// generates a signal build up by the specified function type. v1.6
FUNCTION_BLOCK FB_FunctionGenerator
VAR_INPUT
	bEnable		: BOOL 	:= TRUE;	// set TRUE to generate the specified signal; set FALSE to reset the signal buffer
	fFrequency	: LREAL := 1000;	// in [Hz]
	fAmplitude	: LREAL := 1;
	fOffset		: LREAL	:= 0;	
	nDutyCycle	: UINT 	:= 50;		// in [%] (for pulse function)
	eFunction	: E_FunctionType := E_FunctionType.Sine;	
END_VAR
VAR_IN_OUT
	aSignal		: ARRAY[1..cOversamples] OF LREAL;
END_VAR
VAR_OUTPUT
	bError		: BOOL;
END_VAR

VAR
	bInit						: BOOL := TRUE;
	fbGetTaskIdx				: GETCURTASKINDEX;
	
	fLastFrequency				: LREAL;		// in [Hz]
	fLastAmplitude				: LREAL;
	fLastOffset					: LREAL;
	nLastDutyCycle				: UINT;
	eLastFunction				: E_FunctionType;
	
	nSamples					: UDINT;
	fCycleTime					: LREAL;		// in [s]
	fDelta						: LREAL;		// amplitude delta per sample
	fPhase						: LREAL;		// in [°]
	nSign						: INT := 1;		// 1 or -1
	fLastSignalValue			: LREAL;		// amplitude
	fPeriod						: LREAL;		// in [s]
	fAngularIncrement			: LREAL;		// in [°]
	fAngularIncrementPerCycle	: LREAL;		// in [°]
	fAngularIncrementPerSample	: LREAL;		// in [°]
	(* for modulated signal (carrier signal without offset) *)
	fCarrierFrequency					: LREAL := 500;	// in [Hz] (sine)
	fCarrierAmplitude					: LREAL := 1;
	fCarrierPeriod						: LREAL;		// in [s]
	fCarrierAngularIncrement			: LREAL;		// in [°]
	fCarrierAngularIncrementPerCycle	: LREAL;		// in [°]
	fCarrierAngularIncrementPerSample	: LREAL;		// in [°]
				
END_VAR

IF bEnable THEN
	IF fLastFrequency <> fFrequency THEN
		bInit := TRUE; // For automatic initializing
		fLastFrequency := fFrequency;
	END_IF
	IF fLastAmplitude <> fAmplitude THEN
		bInit := TRUE; // For automatic initializing
		fLastAmplitude := fAmplitude;
	END_IF
	IF fLastOffset <> fOffset THEN
		bInit := TRUE; // For automatic initializing
		fLastOffset := fOffset;
	END_IF
	IF nLastDutyCycle <> nDutyCycle THEN
		bInit := TRUE; // For automatic initializing
		nLastDutyCycle := nDutyCycle;
	END_IF
	IF eLastFunction <> eFunction THEN
		bInit := TRUE; // For automatic initializing
		eLastFunction := eFunction;
	END_IF
	IF bInit THEN
		// Get task info	
		fbGetTaskIdx();
		fCycleTime := UDINT_TO_LREAL(TwinCAT_SystemInfoVarList._TaskInfo[fbGetTaskIdx.index].CycleTime) (*100ns*) / (10.0 * 1000.0 * 1000.0);	
		fLastSignalValue := 0;
		nSign := 1;
		fAngularIncrement := 0;
		// Flush out old data
		MEMSET(ADR(aSignal), 0, SIZEOF(aSignal));
		IF fFrequency > 0 AND fCycleTime > 0 THEN		
			// Calculate period, increments per plc cycle, increment per oversample
			IF cOversamples > 0 THEN			
				IF eFunction = E_FunctionType.Sine THEN
					fPeriod := 1/fFrequency;
					fAngularIncrementPerCycle := 360*(fCycleTime/fPeriod);
					fAngularIncrementPerSample := fAngularIncrementPerCycle/cOversamples;
					// no phase adjustment
					bInit := FALSE;	
				ELSIF eFunction = E_FunctionType.Square	THEN
					fPeriod := 1/fFrequency;
					fAngularIncrementPerCycle  := 360*(fCycleTime/fPeriod);
					fAngularIncrementPerSample := fAngularIncrementPerCycle/cOversamples;
					fPhase := 0.5*360;
					bInit := FALSE;
				ELSIF eFunction = E_FunctionType.Pulse THEN
					fPeriod := 1/fFrequency;
					fAngularIncrementPerCycle  := 360*(fCycleTime/fPeriod);
					fAngularIncrementPerSample := fAngularIncrementPerCycle/cOversamples;
					IF nDutyCycle > 100 THEN
						nDutyCycle := 100;
					END_IF
					fPhase := (UDINT_TO_LREAL(nDutyCycle)/100)*360;
					bInit := FALSE;					
				ELSIF eFunction = E_FunctionType.Triangular THEN
					fPeriod := 1/fFrequency;				
					fAngularIncrementPerCycle  := 360*(fCycleTime/fPeriod);
					fAngularIncrementPerSample := fAngularIncrementPerCycle/cOversamples;
					fPhase := 0.5*360; 
					fDelta := 4*(fAmplitude/(360/fAngularIncrementPerSample));				
					bInit := FALSE;
				ELSIF eFunction = E_FunctionType.Sawtooth THEN
					fPeriod := 1/fFrequency;			
					fAngularIncrementPerCycle  := 360*(fCycleTime/fPeriod);		
					fAngularIncrementPerSample := fAngularIncrementPerCycle/cOversamples;
					fDelta := fAmplitude/(360/fAngularIncrementPerSample);
					bInit := FALSE;
				ELSIF eFunction = E_FunctionType.AM THEN
					fPeriod := 1/fFrequency;
					fAngularIncrementPerCycle := 360*(fCycleTime/fPeriod);
					fAngularIncrementPerSample := fAngularIncrementPerCycle/cOversamples;
					// no phase adjustment
					fCarrierPeriod := 1/fCarrierFrequency;
					fCarrierAngularIncrementPerCycle := 360*(fCycleTime/fCarrierPeriod);
					fCarrierAngularIncrementPerSample := fCarrierAngularIncrementPerCycle/cOversamples;				
					// no phase adjustment	
					bInit := FALSE;
				ELSE
					bError := TRUE;	
				END_IF
			ELSE
				bError := TRUE;
			END_IF
		ELSE
			bError := TRUE;
		END_IF
	END_IF
	
	// Enable function generator
	IF NOT bError THEN		
		CASE eFunction OF		
			// sine: typical for vibrations originating from rotating machine
			E_FunctionType.Sine: Sine();
			
			// square: mixed sine signals good for analyzing spectrum				
			E_FunctionType.Square: Square();
			
			// pulse: mixed sine signals good for analyzing spectrum				
			E_FunctionType.Pulse: Pulse();
	
			// sawtooth: ramp-type vibrations, continuously increasing			
			E_FunctionType.Sawtooth: Sawtooth();
		
			// triangular: mixed sine signals good for analyzing spectrum
			E_FunctionType.Triangular: Triangular();
		
			// amplitude modulation: typical for vibrations originating from gear-tooth failure or bearing faults
			// Carrier signal with own frequency and amplitude		
			E_FunctionType.AM: AM();				
		END_CASE
	END_IF
ELSE
	// Flush out old data
	MEMSET(ADR(aSignal), 0, SIZEOF(aSignal));
	
	bInit := TRUE;
	bError := FALSE;
END_IF

METHOD PRIVATE AM
VAR_INPUT
END_VAR
{warning disable C0371}

FOR nSamples := 1 TO cOversamples DO
	// base signal * carrier signal
	aSignal[nSamples] := ( fAmplitude*SIN(2*PI*(fAngularIncrement+(nSamples-1)*fAngularIncrementPerSample)/360) + fOffset )
							* ( fCarrierAmplitude*SIN(2*PI*(fCarrierAngularIncrement+(nSamples-1)*fCarrierAngularIncrementPerSample)/360) );
END_FOR
// Increment angular positions
fAngularIncrement := fAngularIncrement + fAngularIncrementPerCycle;
fCarrierAngularIncrement := fCarrierAngularIncrement + fCarrierAngularIncrementPerCycle;

{warning restore C0371}
END_METHOD

METHOD PRIVATE Pulse
VAR_INPUT
END_VAR
{warning disable C0371}

FOR nSamples := 1 TO cOversamples DO
	// For pulse wave (unequal phases)
	IF (fAngularIncrement >= 360) THEN
		fAngularIncrement := fAngularIncrement - DINT_TO_LREAL(LREAL_TO_DINT(fAngularIncrement/360))*360;
		// or with Tc2_Math library: fAngularIncrement := LMOD(fAngularIncrement,360);
	END_IF
	IF (fAngularIncrement < fPhase) THEN
		nSign := 1;		
	ELSIF (fAngularIncrement >= fPhase) THEN
		nSign := 0;
	END_IF
	fAngularIncrement := fAngularIncrement + fAngularIncrementPerSample;
	
	aSignal[nSamples] := nSign*fAmplitude;
	
	aSignal[nSamples] := aSignal[nSamples] + fOffset;
END_FOR

{warning restore C0371}
END_METHOD

METHOD PRIVATE Sawtooth
VAR_INPUT
END_VAR
{warning disable C0371}

FOR nSamples := 1 TO cOversamples DO
	// For sawtooth wave (equal phase = period/2)
	IF (fAngularIncrement >= 360) THEN
		fAngularIncrement := fAngularIncrement - DINT_TO_LREAL(LREAL_TO_DINT(fAngularIncrement/360))*360;
		// or with Tc2_Math library: fAngularIncrement := LMOD(fAngularIncrement,360);
		fLastSignalValue := fLastSignalValue -fAmplitude;
	END_IF
	fAngularIncrement := fAngularIncrement + fAngularIncrementPerSample;

	aSignal[nSamples] := fLastSignalValue + fDelta;

	// Store last sample
	fLastSignalValue := aSignal[nSamples];
	
	aSignal[nSamples] := aSignal[nSamples] + fOffset;					
END_FOR	

{warning restore C0371}
END_METHOD

METHOD PRIVATE Sine
VAR_INPUT
END_VAR
{warning disable C0371}

FOR nSamples := 1 TO cOversamples DO
	aSignal[nSamples] := fAmplitude*SIN(2*PI*(fAngularIncrement+(nSamples-1)*fAngularIncrementPerSample)/360);

	aSignal[nSamples] := aSignal[nSamples] + fOffset;
END_FOR

// Increment angular position
fAngularIncrement := fAngularIncrement + fAngularIncrementPerCycle;

{warning restore C0371}
END_METHOD

METHOD PRIVATE Square
VAR_INPUT
END_VAR
{warning disable C0371}

FOR nSamples := 1 TO cOversamples DO
	// For square wave (equal phase = period/2)
	IF (fAngularIncrement >= 360) THEN
		fAngularIncrement := fAngularIncrement - DINT_TO_LREAL(LREAL_TO_DINT(fAngularIncrement/360))*360;
		// or with Tc2_Math library: fAngularIncrement := LMOD(fAngularIncrement,360);
	END_IF
	IF (fAngularIncrement < fPhase) THEN
		nSign := 1;
	ELSIF (fAngularIncrement >= fPhase) THEN
		nSign := -1;
	END_IF
	fAngularIncrement := fAngularIncrement + fAngularIncrementPerSample;
	
	aSignal[nSamples] := nSign*fAmplitude;
	
	aSignal[nSamples] := aSignal[nSamples] + fOffset;
END_FOR

{warning restore C0371}
END_METHOD

METHOD PRIVATE Triangular
VAR_INPUT
END_VAR
{warning disable C0371}

FOR nSamples := 1 TO cOversamples DO
	IF (fAngularIncrement >= 360) THEN
		fAngularIncrement := fAngularIncrement - DINT_TO_LREAL(LREAL_TO_DINT(fAngularIncrement/360))*360;
		// or with Tc2_Math library: fAngularIncrement := LMOD(fAngularIncrement,360);
	END_IF
	// Negative delta -> Positive delta
	IF fAngularIncrement < fPhase/2 THEN	
		nSign := 1;		
	ELSIF fAngularIncrement >= fPhase/2 AND fAngularIncrement < 3*fPhase/2 THEN
		nSign := -1;
	ELSIF fAngularIncrement >= 3*fPhase/2 THEN
		nSign := 1;	
	END_IF
	fAngularIncrement := fAngularIncrement + fAngularIncrementPerSample;
	
	aSignal[nSamples] := fLastSignalValue + nSign*fDelta;
	IF aSignal[nSamples] > fAmplitude THEN
		aSignal[nSamples] := aSignal[nSamples] - 2*(aSignal[nSamples]-fAmplitude);
	ELSIF aSignal[nSamples] < (-1)*fAmplitude THEN
		aSignal[nSamples] := aSignal[nSamples] - 2*(aSignal[nSamples]+fAmplitude);
	END_IF
	
	// Store last sample
	fLastSignalValue := aSignal[nSamples];		
	
	aSignal[nSamples] := aSignal[nSamples] + fOffset;
END_FOR

{warning restore C0371}
END_METHOD

END_FUNCTION_BLOCK
